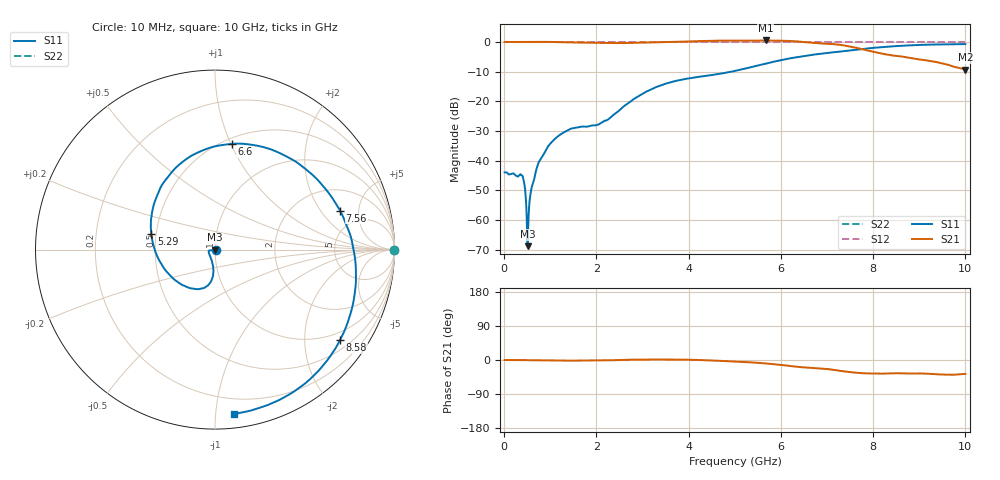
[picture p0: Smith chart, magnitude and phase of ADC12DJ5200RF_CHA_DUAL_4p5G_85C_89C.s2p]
! Texas Instruments, Inc.
! ADC12DJ5200RF - CH A S-Parameters (Dual Ch Mode, Fs = 4.5 GSPS, 85 degC case, 89 degC juntion)
! Port 1 represents the 100-ohm differenal input, Port 2 the digital output
! freq  dbS11  angS11  dbS21 angS21 dbS12 angS12 dbS22 angS22
# HZ S DB R 100
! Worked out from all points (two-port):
!   1000 points, 10 MHz to 10 GHz, reference 100 ohm
!   highest |S21| = 0.52 dB at 5.67 GHz (marker M1); lowest = -9.3 dB at 10 GHz (marker M2)
!   |S21| within 3 dB of the highest: start of sweep to 7.78 GHz
!   lowest |S11| = -68.9 dB at 510 MHz (marker M3), VSWR 1.00, Z = 100 - j0.0713 ohm
!   |S11| at or under -10 dB: start of sweep to 4.932 GHz
!   |S22| runs from 0.0 to 0.0 dB; largest |S21 - S12| = 0.75
!   S11 on the Smith chart (normalised r, x): 10 MHz: 1.01, -0.00; 5.29 GHz: 0.47, +0.10; 6.6 GHz: 0.55, +1.01; 7.56 GHz: 3.35, +3.13; 8.58 GHz: 0.75, -2.91; 10 GHz: 0.09, -1.12
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1e7  -43.98 -7.6  0.00 0.0  0.00 0.0  0.00 0.0
3.8e8  -44.92 -10.5  0.03 -0.3  0.00 0.0  0.00 0.0
4.3e8  -47.24 -0.5  0.03 -0.3  0.00 0.0  0.00 0.0
4.7e8  -52.81 6.8  0.03 -0.4  0.00 0.0  0.00 0.0
5.1e8  -68.87 -81.6  0.03 -0.4  0.00 0.0  0.00 0.0
6e8  -48.82 -136.8  0.04 -0.5  0.00 0.0  0.00 0.0
7.1e8  -42.37 -157.4  0.03 -0.5  0.00 0.0  0.00 0.0
9.4e8  -35.52 -169.1  0.04 -0.9  0.00 0.0  0.00 0.0
1.26e9  -30.80 -171.7  -0.04 -1.6  0.00 0.0  0.00 0.0
1.68e9  -28.56 -163.4  -0.21 -1.5  0.00 0.0  0.00 0.0
2.24e9  -26.25 -119.8  -0.32 -0.9  0.00 0.0  0.00 0.0
3.34e9  -14.98 -96.9  -0.08 1.3  0.00 0.0  0.00 0.0
4.24e9  -11.72 -125.9  0.30 -0.0  0.00 0.0  0.00 0.0
5.01e9  -9.74 -174.4  0.46 -4.4  0.00 0.0  0.00 0.0
5.29e9  -8.74 165.9  0.45 -5.9  0.00 0.0  0.00 0.0
5.67e9  -7.31 140.6  0.52 -9.1  0.00 0.0  0.00 0.0
6.6e9  -4.49 81.1  -0.14 -20.2  0.00 0.0  0.00 0.0
6.67e9  -4.33 76.5  -0.24 -20.9  0.00 0.0  0.00 0.0
7.56e9  -2.73 17.4  -1.71 -32.7  0.00 0.0  0.00 0.0
8.34e9  -1.56 -25.8  -4.34 -35.5  0.00 0.0  0.00 0.0
8.58e9  -1.31 -35.9  -4.82 -35.0  0.00 0.0  0.00 0.0
1e10  -0.71 -83.2  -9.29 -36.6  0.00 0.0  0.00 0.0
